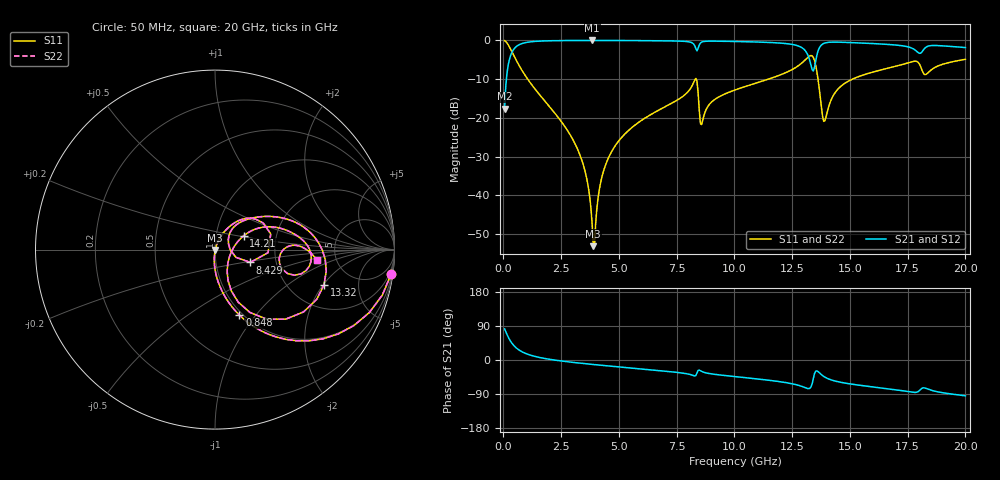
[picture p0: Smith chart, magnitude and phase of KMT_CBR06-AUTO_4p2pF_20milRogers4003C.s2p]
! Data measured by Modelithics Inc. support@modelithics.com 813-866-6335
! KEMET CBR06-AUTO 4.2pF, Pad Width= 0.851mm, Pad Length= 0.64mm, Pad Gap= 0.62mm, 20mil Rogers 4003C substrate Data, January 2022
# hz S ma R 50
! 2 Port Network Data from SP1.SP block
! freq  magS11  angS11  magS21  angS21  magS12  angS12  magS22  angS22
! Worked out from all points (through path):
!   401 points, 50 MHz to 20 GHz, reference 50 ohm
!   highest |S21| = -0.02 dB at 3.841 GHz (marker M1); lowest = -17.6 dB at 50 MHz (marker M2)
!   group delay of S21, straight-line fit = 15.2 ps
!   lowest |S11| = -53.1 dB at 3.89 GHz (marker M3), VSWR 1.00, Z = 50.2 - j0.162 ohm
!   |S11| at or under -10 dB: 1.049 GHz to 8.309 GHz (7.26 GHz wide, 155 % of centre); 8.341 GHz to 11.47 GHz (3.129 GHz wide, 31.6 % of centre); 13.62 GHz to 15.11 GHz (1.49 GHz wide, 10.4 % of centre)
!   |S22| runs from -53.1 to -0.1 dB; largest |S21 - S12| = 0
!   S11 on the Smith chart (normalised r, x): 50 MHz: 1, -15; 848 MHz: 0.96, -0.83; 8.429 GHz: 1.47, -0.22; 13.32 GHz: 3.07, -2.04; 14.21 GHz: 1.36, +0.22; 20 GHz: 3.54, -0.60
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5e7  0.9912 -7.7  0.1318 82.3  0.1318 82.3  0.9912 -7.7
2.99375e8  0.7802 -39.6  0.6246 50.4  0.6246 50.4  0.7802 -39.6
8.48e8  0.3896 -69.5  0.9199 20.3  0.9199 20.3  0.3896 -69.5
3.391625e9  0.02854 -95.4  0.9978 -8.8  0.9978 -8.8  0.02854 -95.4
3.641e9  0.01455 -93.5  0.998 -10.4  0.998 -10.4  0.01455 -93.5
3.8405e9  0.004246 -76.5  0.9981 -11.6  0.9981 -11.6  0.004246 -76.5
3.890375e9  0.002212 -47.0  0.9981 -11.9  0.9981 -11.9  0.002212 -47.0
4.2395e9  0.01616 69.3  0.9978 -14.0  0.9978 -14.0  0.01616 69.3
4.688375e9  0.03698 70.4  0.9972 -16.5  0.9972 -16.5  0.03698 70.4
6.73325e9  0.1265 60.8  0.9889 -27.9  0.9889 -27.9  0.1265 60.8
8.279375e9  0.307 28.8  0.8564 -42.2  0.8564 -42.2  0.307 28.8
8.429e9  0.2091 -19.9  0.792 -27.3  0.792 -27.3  0.2091 -19.9
8.6285e9  0.09387 37.6  0.9622 -31.4  0.9622 -31.4  0.09387 37.6
1.0025e10  0.2292 45.0  0.9683 -43.8  0.9683 -43.8  0.2292 45.0
1.271825e10  0.4602 20.2  0.8567 -65.9  0.8567 -65.9  0.4602 20.2
1.331675e10  0.6382 -18.0  0.4757 -71.0  0.4757 -71.0  0.6382 -18.0
1.336662e10  0.6309 -26.1  0.4188 -62.4  0.4188 -62.4  0.6309 -26.1
1.386538e10  0.09019 -27.9  0.9123 -43.3  0.9123 -43.3  0.09019 -27.9
1.42145e10  0.1781 25.8  0.9496 -53.0  0.9496 -53.0  0.1781 25.8
1.670825e10  0.4425 12.0  0.8845 -76.5  0.8845 -76.5  0.4425 12.0
1.805488e10  0.4651 -17.9  0.6823 -77.9  0.6823 -77.9  0.4651 -17.9
2e10  0.5702 -5.8  0.8084 -94.5  0.8084 -94.5  0.5702 -5.8
